VAR_GLOBAL
	LON_IN_1 	AT %I*:ST_LON_Parameter_IN_36B;
	LON_OUT_1 	AT %Q*:ST_LON_Parameter_OUT_36B;
	stLON_Com_1	: ST_LON_Communication;

	LON_IN_2 	AT %I*:ST_LON_Parameter_IN_36B;
	LON_OUT_2 	AT %Q*:ST_LON_Parameter_OUT_36B;
	stLON_Com_2	: ST_LON_Communication;

	LON_IN_3 	AT %I*:ST_LON_Parameter_IN_36B;
	LON_OUT_3 	AT %Q*:ST_LON_Parameter_OUT_36B;
	stLON_Com_3	: ST_LON_Communication;

	LON_IN_4 	AT %I*:ST_LON_Parameter_IN_36B;
	LON_OUT_4 	AT %Q*:ST_LON_Parameter_OUT_36B;
	stLON_Com_4	: ST_LON_Communication;

	LON_IN_5 	AT %I*:ST_LON_Parameter_IN_36B;
	LON_OUT_5 	AT %Q*:ST_LON_Parameter_OUT_36B;
	stLON_Com_5	: ST_LON_Communication;

	LON_IN_6 	AT %I*:ST_LON_Parameter_IN_36B;
	LON_OUT_6 	AT %Q*:ST_LON_Parameter_OUT_36B;
	stLON_Com_6	: ST_LON_Communication;

	LON_IN_7 	AT %I*:ST_LON_Parameter_IN_36B;
	LON_OUT_7 	AT %Q*:ST_LON_Parameter_OUT_36B;
	stLON_Com_7	: ST_LON_Communication;
END_VAR
